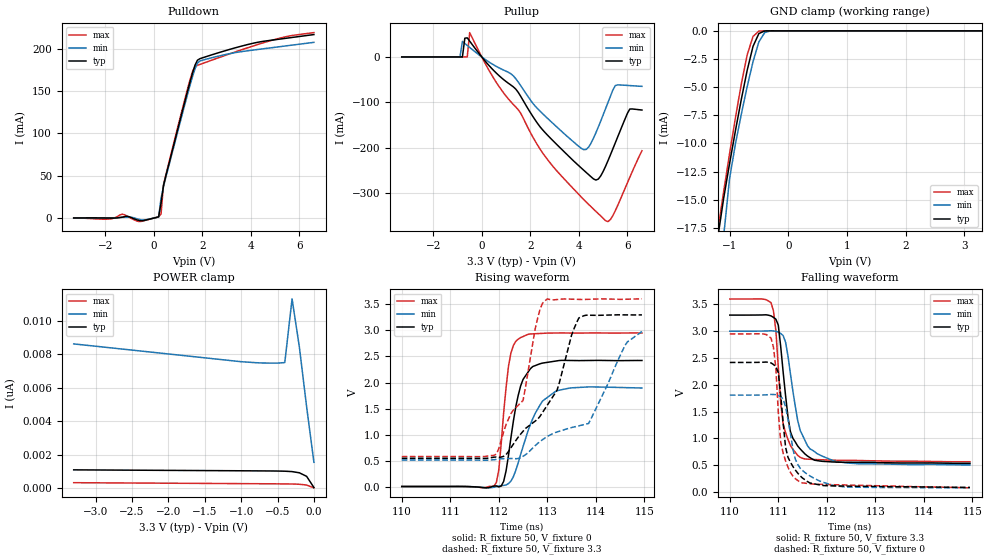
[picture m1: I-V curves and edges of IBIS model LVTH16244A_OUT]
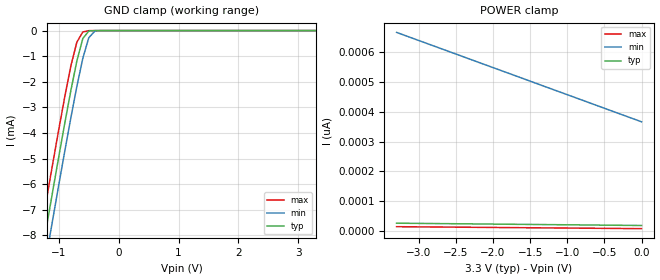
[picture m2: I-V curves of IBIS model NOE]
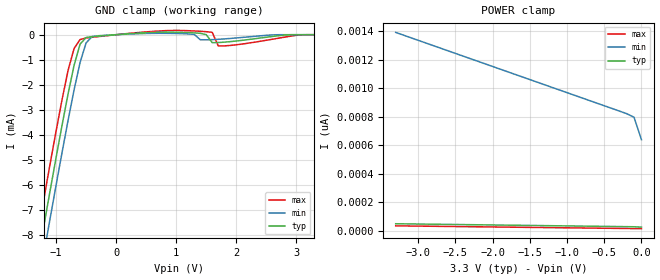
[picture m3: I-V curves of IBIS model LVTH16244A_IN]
|   TEXAS INSTRUMENTS INCORPORATED
|   Standard Linear and Logic
|   IBIS Model of SN74LVTH16244ADGGR
|   3.3V ABT OCTAL  BUFFER/DRIVERS with 3-STATE OUTPUTS
|   TSSOP 48 PIN PACKAGE (DGGR)
[IBIS Ver]   2.1
[Comment char]   |_char
[File Name]   h16244a.ibs
[File Rev]   1.0
[Date]   04-20-2000
[Source]   Data created from HSPICE simulations at TI ,SLL.
[Notes]   The following is an IBIS list for LVTH16244A
   - All test data contained in this file are derived from hspice
   (tm) simulations.
   - File created by Moshiul Haque, SLL applications.
|   -For Questions or Comments please E-mailto:  sllibis@ti.com
|  [Disclaimer]
|*   Property of Texas Instruments Incorporated.  Unauthorized   *
|*   reproduction and/or distribution is strictly prohibited.   *
|*   This product is protected under copyright law.   *
|*   Created 1995, (C) Copyright 1995, Texas Instruments Inc.,   *
|*   All Rights Reserved   *
|*   UNLESS THERE IS A SIGNED, WRITTEN AGREEMENT TO THE   *
|*   CONTRARY, TEXAS INSTRUMENTS ("TI") IS PROVIDING THE SPICE   *
|*   MODELS "AS IS" AND WITHOUT ANY WARRANTY, EXPRESSED OR   *
|*   IMPLIED.  TI assumes no liability for:   *
|*   1) the accuracy of the IBIS models provided to your   *
|*   company;   *
|*   2) the proper functioning of these IBIS models in your   *
|*   design or for any resulting applications; or   *
|*   3) infringement of patents, copyrights or intellectual   *
|*   property rights resulting from your use of these   *
|*   IBIS models.   *
|*   TI provides IBIS Models as a service to our customers.   *
|*   You and your company shall not distribute, sell or give   *
|*   these models to anyone else without prior written   *
|*   permission from TI.   *
|*   TI reserves the right to make changes to our products or   *
|*   to discontinue any semiconductor product or service   *
|*   without notice, and advises our customers to obtain the   *
|*   latest version of relevant information to verify, before   *
|*   placing orders, that the information being relied on is   *
|*   current.   *
|*   Please be aware that your receipt and use of the IBIS   *
|*   information provided shall serve as acceptance of these   *
|*   terms and conditions.  If you do not accept these terms,   *
|*   you should return or destroy the IBIS models and any   *
|*   other accompanying information immediately.   *
[Component]   LVTH16244A
[manufacturer]   Texas Instruments, Inc.
[Package]
|   typ   min   max
R_pkg   0.04   0.035   0.051
L_pkg   3.49nH   3.035nH   4.314nH
C_pkg   0.42pF   0.346pF   0.502pF
[Pin]   signal_name   model_name   R_pin   L_pin   C_pin
1   1N0E   NOE   0.039   3.987nH   0.654pF
2   1Y1   LVTH16244A_OUT   0.047   3.725nH   0.659pF
3   1Y2   LVTH16244A_OUT   0.059   3.692nH   0.604pF
4   GND   GND   0.068   3.675nH   0.606pF
5   1Y3   LVTH16244A_OUT   0.055   3.473nH   0.547pF
6   1Y4   LVTH16244A_OUT   0.056   3.402nH   0.497pF
7   VCC   POWER   0.057   3.3nH   0.492pF
8   2Y1   LVTH16244A_OUT   0.056   3.189nH   0.455pF
9   2Y2   LVTH16244A_OUT   0.058   3.154nH   0.449pF
10   GND   GND   0.058   3.094nH   0.436pF
11   2Y3   LVTH16244A_OUT   0.058   3.078nH   0.424pF
12   2Y4   LVTH16244A_OUT   0.06   3.081nH   0.414pF
13   3Y1   LVTH16244A_OUT   0.061   3.097nH   0.416pF
14   3Y2   LVTH16244A_OUT   0.06   3.126nH   0.427pF
15   GND   GND   0.061   3.158nH   0.44pF
16   3Y3   LVTH16244A_OUT   0.058   3.173nH   0.45pF
17   3Y4   LVTH16244A_OUT   0.056   3.189nH   0.455pF
18   VCC   POWER   0.056   3.265nH   0.49pF
19   4Y1   LVTH16244A_OUT   0.054   3.322nH   0.492pF
20   4Y2   LVTH16244A_OUT   0.052   3.388nH   0.544pF
21   GND   GND   0.064   3.591nH   0.605pF
22   4Y3   LVTH16244A_OUT   0.059   3.677nH   0.612pF
23   4Y4   LVTH16244A_OUT   0.046   3.678nH   0.668pF
24   4NOE   NOE   0.041   3.979nH   0.659pF
25   3NOE   NOE   0.04   3.995nH   0.658pF
26   4A4   LVTH16244A_IN   0.046   3.69nH   0.662pF
27   4A3   LVTH16244A_IN   0.057   3.649nH   0.602pF
28   GND   GND   0.066   3.615nH   0.602pF
29   4A2   LVTH16244A_IN   0.055   3.447nH   0.547pF
30   4A1   LVTH16244A_IN   0.054   3.326nH   0.492pF
31   VCC   POWER   0.055   3.239nH   0.488pF
32   3A4   LVTH16244A_IN   0.056   3.183nH   0.454pF
33   3A3   LVTH16244A_IN   0.057   3.144nH   0.447pF
34   GND   GND   0.058   3.099nH   0.436pF
35   3A2   LVTH16244A_IN   0.059   3.086nH   0.425pF
36   3A1   LVTH16244A_IN   0.06   3.081nH   0.414pF
37   2A4   LVTH16244A_IN   0.061   3.097nH   0.415pF
38   2A3   LVTH16244A_IN   0.06   3.119nH   0.427pF
39   GND   GND   0.06   3.144nH   0.439pF
40   2A2   LVTH16244A_IN   0.056   3.13nH   0.446pF
41   2A1   LVTH16244A_IN   0.057   3.208nH   0.456pF
42   VCC   POWER   0.056   3.247nH   0.487pF
43   1A4   LVTH16244A_IN   0.054   3.328nH   0.491pF
44   1A3   LVTH16244A_IN   0.053   3.413nH   0.546pF
45   GND   GND   0.066   3.609nH   0.606pF
46   1A2   LVTH16244A_IN   0.058   3.689nH   0.607pF
47   1A1   LVTH16244A_IN   0.047   3.727nH   0.662pF
48   2NOE   NOE   0.04   3.978nH   0.655pF
| Models and submodels in the file (3): LVTH16244A_OUT (3-state), NOE (Input), LVTH16244A_IN (Input)
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|   Model LVTH16244A  OUTPUT
[Model]   LVTH16244A_OUT
|Signals
Model_type  3-state
Polarity   Inverting
Enable   Active-Low
Vmeas= 1.5V
Cref = 50pf
Rref = 500
Vref = 0V
| variable   typ   min   max
C_comp   0.3p   NA   NA
[Temperature Range]   50   100   0
[Voltage range]   3.3   3   3.6
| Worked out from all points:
|   slope of the pulldown table from 0 to 0.495 V, typ, clamps not added: 10 ohm
|   slope of the pullup table from 0 to 0.495 V, typ, clamps not added: 16.5 ohm
|   GND clamp passes 1 mA (typ) near -0.57 V on its own axis
|   rising waveform, R_fixture 50, V_fixture 0: 20-80 % time 271ps typ, 444ps min, 183ps max; typ from 0.006 V to 2.42 V
|   falling waveform, R_fixture 50, V_fixture 3.3: 20-80 % time 220ps typ, 323ps min, 178ps max; typ from 3.3 V to 0.535 V
|   rising waveform, R_fixture 50, V_fixture 3.3: 20-80 % time 927ps typ, 1.4ns min, 598ps max; typ from 0.546 V to 3.3 V
|   falling waveform, R_fixture 50, V_fixture 0: 20-80 % time 220ps typ, 297ps min, 185ps max; typ from 2.42 V to 0.087 V
|Process range|   weak   strong
[Pullup]
|   50C:3.3V:   100C:3V:weak   0C:3.6V:strong
|   Voltage   I(typ)   I(min)   I(max)
-3.3V     70.42uA    59uA       80.74uA
-900mV    69.34uA    46.54uA    79.72uA
-800mV    63.71uA    34.29mA    79.65uA
-600mV    42.05mA    25.32mA    54.7uA
-500mV    34.8mA     20.93mA    53.67mA
2.5V      -159.8mA   -124.4mA   -210.4mA
4.2V      -249mA     -203.9mA   -313.5mA
4.7V      -270.6mA   -166.9mA   -339.4mA
5.1V      -240.4mA   -113.8mA   -360mA
5.5V      -189mA     -62.98mA   -338.3mA
6.1V      -114.5mA   -62.89mA   -264.5mA
6.6V      -116.7mA   -64.65mA   -206.2mA
[Pulldown]
|   50C:3.3V:   100C:3V:weak   0C:3.6V:strong
|   Voltage   I(typ)   I(min)   I(max)
-3.3V     38.2uA     84.3uA     -26.3uA
-1.8V     -125.3uA   212.3uA    -1.147mA
-1.3V     945.5uA    699uA      4.491mA
-600mV    -3.071mA   -1.706mA   -4.224mA
200mV     1.37mA     1.325mA    1.431mA
300mV     17.54mA    23.27mA    4.721mA
400mV     38.17mA    36.88mA    39.25mA
1.4V      150.5mA    146.8mA    153.2mA
1.6V      171.4mA    167.2mA    173.1mA
1.9V      188mA      185.3mA    181.2mA
4.2V      206.9mA    198.6mA    204mA
6.6V      216.5mA    207.3mA    218.9mA
[GND Clamp]
|   50C:3.3V:   100C:3V:weak   0C:3.6V:strong
|   Voltage   I(typ)   I(min)   I(max)
-3.3V     -662mA     -678mA     -636.5mA
-1.2V     -18.38mA   -28.13mA   -17.77mA
-1.1V     -14.88mA   -18.25mA   -14.27mA
-1V       -11.81mA   -13.15mA   -10.94mA
-900mV    -8.89mA    -10.05mA   -7.747mA
-800mV    -6.107mA   -7.421mA   -4.744mA
-700mV    -3.525mA   -4.972mA   -2.153mA
-600mV    -1.383mA   -2.744mA   -502.1uA
-500mV    -239uA     -981uA     -22.49uA
-400mV    -11.4uA    -147.9uA   -443.1nA
-300mV    -355nA     -8.958uA   -13.48nA
3.3V      56.69pA    11.31nA    -1.707nA
[POWER Clamp]
|   50C:3.3V:   100C:3V:weak   0C:3.6V:strong
|   Voltage   I(typ)   I(min)   I(max)
-3.3V     1.109nA    8.624nA    343.3pA
-1V       1.054nA    7.562nA    287.6pA
-700mV    1.046nA    7.485nA    279.9pA
-400mV    1.029nA    7.511nA    271.1pA
-300mV    1.005nA    11.31nA    265.1pA
-200mV    934.4pA    8.447nA    249.9pA
-100mV    721.8pA    4.869nA    202pA
0V        56.69pA    1.561nA    35.74pA
[ramp]
| variable   typ   min   max
dV/dt_r   1.9316E+00/2.2071E-10  1.7064E+00/3.3159E-10  2.1097E+00/1.3401E-10
dV/dt_f   1.6631E+00/3.9278E-10  1.5039E+00/3.8019E-10  1.8216E+00/3.3992E-10
[Rising Waveform]
R_fixture = 50
V_fixture = 0
V_fixture_min = 0
V_fixture_max = 0
C_fixture = 0pf
L_fixture=0nH
|   50C:3.3V:   100C:3V:weak   0C:3.6V:strong
|   Time   V(typ)   V(min)   V(max)
110ns     5.716mV    5.195mV    6.162mV
111.9ns   14.35mV    -8.536mV   11.99mV
112ns     -2.174mV   12.76mV    323.9mV
112.1ns   103mV      26.76mV    1.42V
112.2ns   605mV      62.38mV    2.314V
112.4ns   1.753V     459.4mV    2.833V
112.5ns   2.059V     771.3mV    2.882V
112.8ns   2.324V     1.409V     2.936V
113.2ns   2.408V     1.817V     2.949V
114.9ns   2.422V     1.895V     2.95V
[Falling Waveform]
R_fixture = 50
V_fixture = 3.3
V_fixture_min = 3
V_fixture_max = 3.6
C_fixture = 0pf
L_fixture=0nH
|   50C:3.3V:   100C:3V:weak   0C:3.6V:strong
|   Time   V(typ)   V(min)   V(max)
110ns     3.3V       3V         3.6V
110.9ns   3.285V     3.008V     3.531V
110.9ns   3.224V     2.998V     3.01V
111ns     3.112V     2.981V     2.324V
111.1ns   2.233V     2.918V     1.264V
111.2ns   1.125V     2.204V     868mV
111.4ns   805mV      1.152V     648mV
111.6ns   644mV      807mV      612mV
112.2ns   558mV      569mV      593mV
114.9ns   535mV      506mV      566mV
[Rising Waveform]
R_fixture = 50
V_fixture = 3.3
V_fixture_min = 3
V_fixture_max = 3.6
C_fixture = 0pf
L_fixture=0nH
|   50C:3.3V:   100C:3V:weak   0C:3.6V:strong
|   Time   V(typ)   V(min)   V(max)
110ns     545.7mV    512.7mV    579.6mV
112ns     570.9mV    525mV      628.1mV
112.3ns   748.7mV    543.2mV    1.405V
112.5ns   1.065V     585.1mV    1.656V
112.9ns   1.424V     902.3mV    3.518V
113.2ns   1.851V     1.051V     3.591V
113.6ns   3.141V     1.158V     3.595V
113.9ns   3.291V     1.214V     3.596V
114.6ns   3.297V     2.711V     3.596V
114.9ns   3.297V     2.978V     3.603V
[Falling Waveform]
R_fixture = 50
V_fixture = 0
V_fixture_min = 0
V_fixture_max = 0
C_fixture = 0pf
L_fixture=0nH
|   50C:3.3V:   100C:3V:weak   0C:3.6V:strong
|   Time   V(typ)   V(min)   V(max)
110ns     2.417V     1.808V     2.95V
110.9ns   2.408V     1.821V     2.87V
110.9ns   2.34V      1.816V     2.297V
111ns     2.227V     1.802V     1.487V
111.1ns   1.802V     1.777V     933mV
111.1ns   833mV      1.588V     582mV
111.4ns   412mV      615mV      250mV
111.4ns   303mV      446mV      184mV
112.3ns   112mV      98.2mV     133mV
114.9ns   87.4mV     80.2mV     79mV
|   LVTH16244A NOE
[Model]   NOE
|Signals
Model_type  Input
Polarity   Non-Inverting
Vinl = 0.8V
Vinh = 2.0V
| variable   typ   min   max
C_comp   0.3p   NA   NA
[Temperature Range]   50   100   0
[Voltage range]   3.3   3   3.6
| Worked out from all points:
|   GND clamp passes 1 mA (typ) near -0.68 V on its own axis
|Process range|   weak   strong
[GND Clamp]
|   50C:3.3V:   100C:3V:weak   0C:3.6V:strong
|   Voltage   I(typ)   I(min)   I(max)
-3.3V     -36.95mA   -38.01mA   -35.9mA
-1.3V     -8.944mA   -10.05mA   -7.862mA
-1.2V     -7.582mA   -8.693mA   -6.503mA
-1.1V     -6.233mA   -7.342mA   -5.159mA
-900mV    -3.6mA     -4.691mA   -2.565mA
-800mV    -2.345mA   -3.409mA   -1.382mA
-700mV    -1.19mA    -2.185mA   -453.1uA
-600mV    -309.3uA   -1.081mA   -54.51uA
-500mV    -19.64uA   -278uA     -2.59uA
-400mV    -750.2nA   -21.97uA   -121.9nA
3.3V      18.56pA    393.3pA    7.338pA
[POWER Clamp]
|   50C:3.3V:   100C:3V:weak   0C:3.6V:strong
|   Voltage   I(typ)   I(min)   I(max)
-3.3V     26.26pA    665.7pA    14.57pA
-1.6V     22.3pA     511.4pA    11.15pA
-800mV    20.43pA    438.7pA    9.547pA
0V        18.56pA    366.1pA    7.94pA
|   LVTH16244A INPUT
[Model]   LVTH16244A_IN
| Signals
Model_type  Input
Vinl = 0.8V
Vinh = 2.0V
| variable   typ   min   max
C_comp   0.3p   NA   NA
[Temperature Range]   50   100   0
[Voltage range]   3.3   3   3.6
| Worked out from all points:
|   GND clamp passes 1 mA (typ) near -0.67 V on its own axis
|Process range|   weak   strong
[GND Clamp]
|   50C:3.3V:   100C:3V:weak   0C:3.6V:strong
|   Voltage   I(typ)   I(min)   I(max)
-3.3V     -36.95mA   -38.02mA   -35.9mA
-1.3V     -8.951mA   -10.06mA   -7.871mA
-1.2V     -7.59mA    -8.699mA   -6.513mA
-1.1V     -6.242mA   -7.35mA    -5.172mA
-800mV    -2.365mA   -3.423mA   -1.425mA
-700mV    -1.223mA   -2.204mA   -552uA
-600mV    -376.8uA   -1.11mA    -193.1uA
-500mV    -112.6uA   -327.6uA   -130.3uA
-300mV    -58.01uA   -41.81uA   -77.25uA
1.5V      1.985uA    -203.1uA   119.7uA
1.8V      -297.4uA   -168uA     -446.8uA
3.3V      26.05pA    839.6pA    -971.7pA
[POWER Clamp]
|   50C:3.3V:   100C:3V:weak   0C:3.6V:strong
|   Voltage   I(typ)   I(min)   I(max)
-3.3V     49.59pA    1.39nA     34.84pA
-200mV    29.12pA    820.9pA    16.31pA
-100mV    28.41pA    795.8pA    15.73pA
0V        26.05pA    638.2pA    15.14pA
